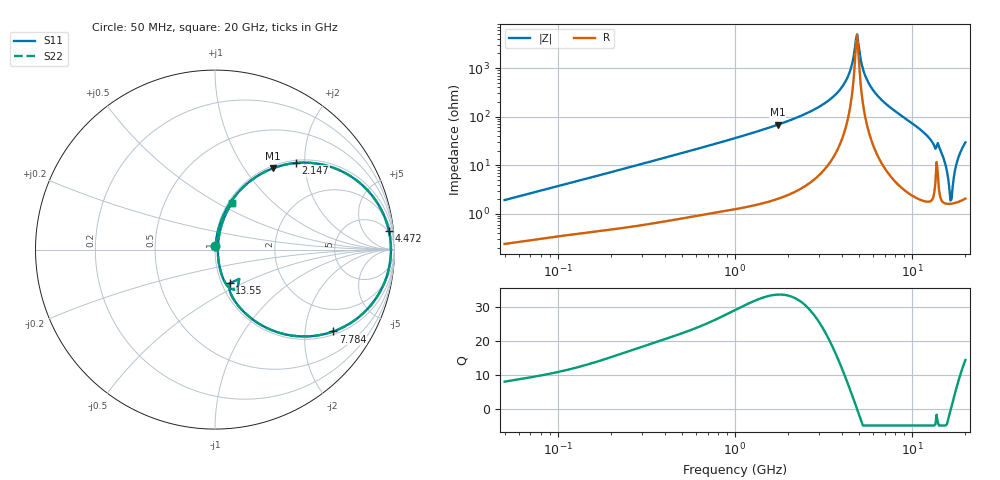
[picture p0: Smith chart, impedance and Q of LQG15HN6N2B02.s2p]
!Murata Part Number: LQG15HN6N2B02
!These Parameters are Measured in Series Mode Connection
!  o--[Z]--o
!Port1  Port2
!  o-------o
!Freq. Start=50[MHz] Stop=20[GHz], 401[Steps]
# Hz S RI R 50
!Freq.(Hz) S11(Real) S11(Imag) S21(Real) S21(Imag) S12(Real) S12(Imag) S22(Real) S22(Imag)
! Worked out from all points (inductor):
!   401 points, 50 MHz to 20 GHz, reference 50 ohm
!   read as one part in series: L = 5.98 nH near 51.52 MHz
!   highest Q = 33.6 at 1.741 GHz (marker M1), where L = 6.22 nH
!   self-resonance near 4.82 GHz
!   S11 on the Smith chart (normalised r, x): 50 MHz: 1.00, +0.04; 2.147 GHz: 1.06, +1.80; 4.472 GHz: 4, +17; 7.784 GHz: 1.10, -2.81; 13.55 GHz: 1.09, -0.43; 20 GHz: 1.04, +0.59
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5e7  0.00275 0.0189  0.9973 -0.0189  0.9973 -0.0189  0.00275 0.0189
1.364002e8  0.00638 0.0491  0.9936 -0.0491  0.9936 -0.0491  0.00638 0.0491
3.721004e8  0.0235 0.1283  0.9765 -0.1283  0.9765 -0.1283  0.0235 0.1283
1e9  0.1233 0.312  0.8767 -0.312  0.8767 -0.312  0.1233 0.312
1.740566e9  0.3214 0.4524  0.6786 -0.4524  0.6786 -0.4524  0.3214 0.4524
2.146657e9  0.4505 0.4825  0.5495 -0.4825  0.5495 -0.4825  0.4505 0.4825
2.728004e9  0.6352 0.464  0.3648 -0.464  0.3648 -0.464  0.6352 0.464
3.736399e9  0.8833 0.2909  0.1167 -0.2909  0.1167 -0.2909  0.8833 0.2909
4.472136e9  0.9688 0.1053  0.0312 -0.1053  0.0312 -0.1053  0.9688 0.1053
4.748272e9  0.9792 0.0335  0.0208 -0.0335  0.0208 -0.0335  0.9792 0.0335
4.89267e9  0.9803 -0.00329  0.0197 0.00329  0.0197 0.00329  0.9803 -0.00329
5.273168e9  0.9707 -0.0962  0.0293 0.0962  0.0293 0.0962  0.9707 -0.0962
5.683258e9  0.9428 -0.1869  0.0572 0.1869  0.0572 0.1869  0.9428 -0.1869
7.442007e9  0.7113 -0.4337  0.2887 0.4337  0.2887 0.4337  0.7113 -0.4337
7.784049e9  0.6589 -0.456  0.3411 0.456  0.3411 0.456  0.6589 -0.456
1.034674e10  0.3139 -0.4479  0.6861 0.4479  0.6861 0.4479  0.3139 -0.4479
1.354865e10  0.0819 -0.1876  0.9181 0.1876  0.9181 0.1876  0.0819 -0.1876
1.504638e10  0.0344 -0.131  0.9656 0.131  0.9656 0.131  0.0344 -0.131
1.646126e10  0.0159 -0.00947  0.9841 0.00947  0.9841 0.00947  0.0159 -0.00947
1.696185e10  0.0171 0.0319  0.9829 -0.0319  0.9829 -0.0319  0.0171 0.0319
1.828096e10  0.0367 0.1368  0.9633 -0.1368  0.9633 -0.1368  0.0367 0.1368
2e10  0.0954 0.2609  0.9046 -0.2609  0.9046 -0.2609  0.0954 0.2609
